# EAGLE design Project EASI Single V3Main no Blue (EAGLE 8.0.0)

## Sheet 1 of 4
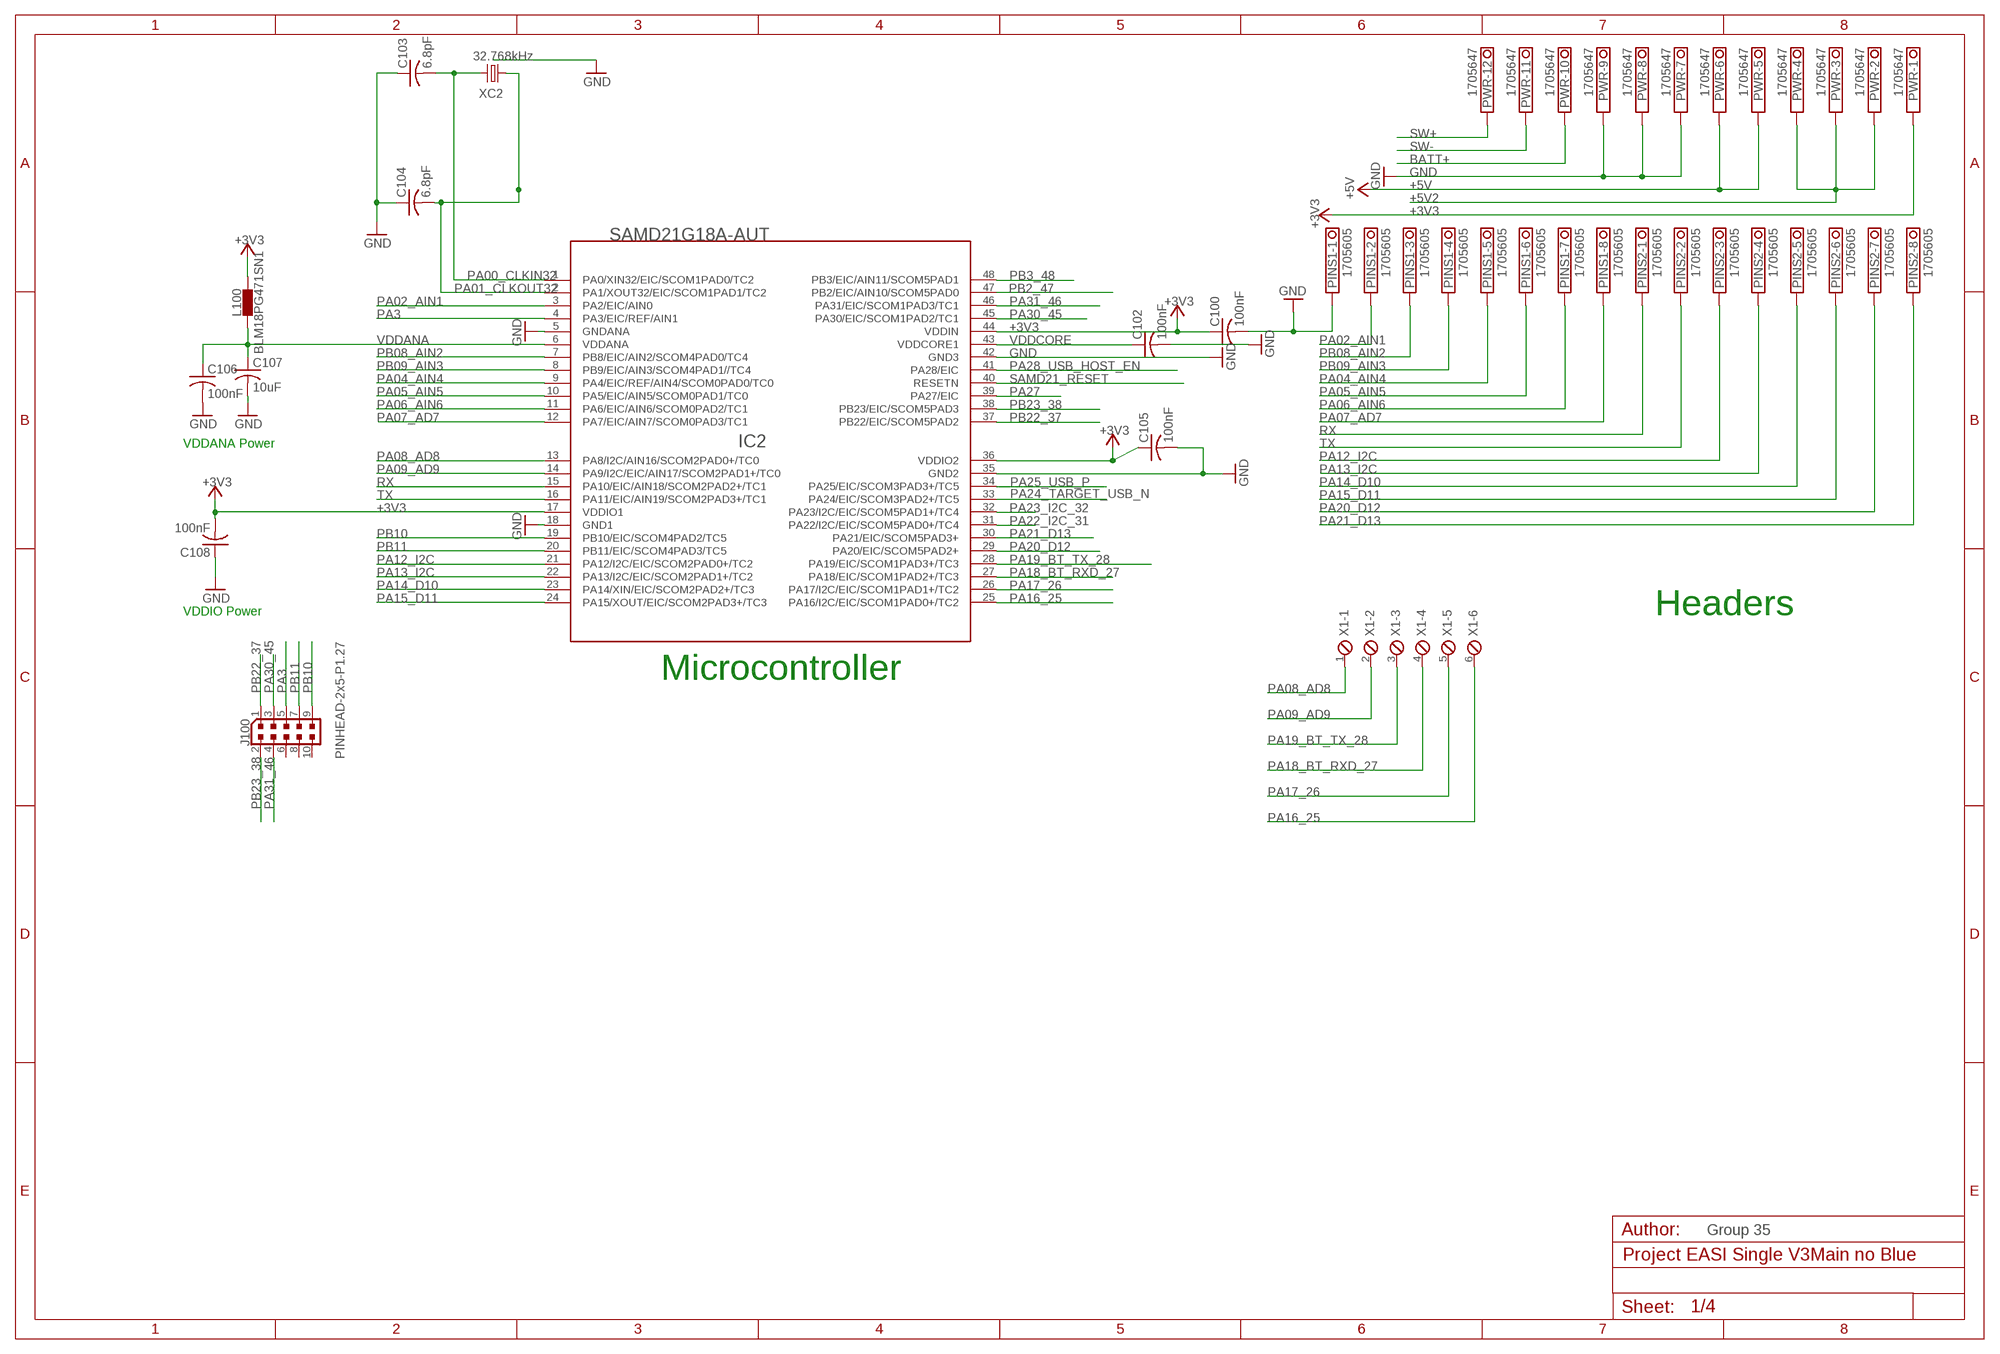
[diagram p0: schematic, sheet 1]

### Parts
C100  100nF  C-USC0805  [C0805]
C102  100nF  C-USC0805  [C0805]
C103  6.8pF  C-USC0805  [C0805]
C104  6.8pF  C-USC0805  [C0805]
C105  100nF  C-USC0805  [C0805]
C106  100nF  C-USC0805  [C0805]
C107  10uF  C-USC0805  [C0805]
C108  100nF  C-USC0805  [C0805]
IC2  SAMD21G18A-AUT  SAMD21G18A  [TQFP48]
J100  PINHEAD-2x5-P1.27  0171_PH127-205DF055G00AROUND-PADS  [PINHEAD_2X05_127]
L100  BLM18PG471SN1  INDUCTOR-0603  [C0603]
PINS1  1705605  [1705605]
PINS2  1705605  [1705605]
PWR  1705647  [1705647]
X1  MPT6  [6POL254]
XC2  32.768kHz  CRYSTALSMD  [CRYSTAL_TC26SMD]

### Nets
+3V3: C100.1 C105.1 C108.2 IC2.17(VDDIO1) IC2.36(VDDIO2) IC2.44(VDDIN) L100.2 PWR.1.1 PWR.1.2 ; also sheet 3
+5V: PWR.5.1 PWR.5.2 PWR.6.1 PWR.6.2 ; also sheet 3
+5V2: PWR.2.1 PWR.2.2 PWR.3.1 PWR.3.2 PWR.4.1 PWR.4.2 ; also sheet 3
BATT+: PWR.10.1 PWR.10.2 ; also sheet 3
GND [gnd]: C100.2 C102.2 C103.1 C104.1 C105.2 C106.2 C107.2 C108.1 IC2.5(GNDANA) IC2.18(GND1) IC2.35(GND2) IC2.42(GND3) PINS1.1.1 PINS1.1.2 PWR.7.1 PWR.7.2 PWR.8.1 PWR.8.2 PWR.9.1 PWR.9.2 XC2.P$1(GND) ; also sheet 3
PA00_CLKIN32: C103.2 IC2.1(PA0/XIN32/EIC/SCOM1PAD0/TC2) XC2.2
PA01_CLKOUT32: C104.2 IC2.2(PA1/XOUT32/EIC/SCOM1PAD1/TC2) XC2.1
PA02_AIN1: IC2.3(PA2/EIC/AIN0) PINS1.2.1 PINS1.2.2
PA3: IC2.4(PA3/EIC/REF/AIN1) J100.5 ; also sheet 2
PA04_AIN4: IC2.9(PA4/EIC/REF/AIN4/SCOM0PAD0/TC0) PINS1.5.1 PINS1.5.2
PA05_AIN5: IC2.10(PA5/EIC/AIN5/SCOM0PAD1/TC0) PINS1.6.1 PINS1.6.2
PA06_AIN6: IC2.11(PA6/EIC/AIN6/SCOM0PAD2/TC1) PINS1.7.1 PINS1.7.2
PA07_AD7: IC2.12(PA7/EIC/AIN7/SCOM0PAD3/TC1) PINS1.8.1 PINS1.8.2
PA08_AD8: IC2.13(PA8/I2C/AIN16/SCOM2PAD0+/TC0) X1.1
PA09_AD9: IC2.14(PA9/I2C/EIC/AIN17/SCOM2PAD1+/TC0) X1.2
PA12_I2C: IC2.21(PA12/I2C/EIC/SCOM2PAD0+/TC2) PINS2.3.1 PINS2.3.2
PA13_I2C: IC2.22(PA13/I2C/EIC/SCOM2PAD1+/TC2) PINS2.4.1 PINS2.4.2
PA14_D10: IC2.23(PA14/XIN/EIC/SCOM2PAD2+/TC3) PINS2.5.1 PINS2.5.2
PA15_D11: IC2.24(PA15/XOUT/EIC/SCOM2PAD3+/TC3) PINS2.6.1 PINS2.6.2
PA16_25: IC2.25(PA16/I2C/EIC/SCOM1PAD0+/TC2) X1.6
PA17_26: IC2.26(PA17/I2C/EIC/SCOM1PAD1+/TC2) X1.5
PA18_BT_RXD_27: IC2.27(PA18/EIC/SCOM1PAD2+/TC3) X1.4
PA19_BT_TX_28: IC2.28(PA19/EIC/SCOM1PAD3+/TC3) X1.3
PA20_D12: IC2.29(PA20/EIC/SCOM5PAD2+) PINS2.7.1 PINS2.7.2
PA21_D13: IC2.30(PA21/EIC/SCOM5PAD3+) PINS2.8.1 PINS2.8.2
PA22_I2C_31: IC2.31(PA22/I2C/EIC/SCOM5PAD0+/TC4) ; also sheet 2
PA23_I2C_32: IC2.32(PA23/I2C/EIC/SCOM5PAD1+/TC4) ; also sheet 2
PA24_TARGET_USB_N [USBpair]: IC2.33(PA24/EIC/SCOM3PAD2+/TC5)
PA25_USB_P [USBpair]: IC2.34(PA25/EIC/SCOM3PAD3+/TC5)
PA27: IC2.39(PA27/EIC)
PA28_USB_HOST_EN: IC2.41(PA28/EIC)
PA30_45: IC2.45(PA30/EIC/SCOM1PAD2/TC1) J100.3 ; also sheet 2
PA31_46: IC2.46(PA31/EIC/SCOM1PAD3/TC1) J100.4 ; also sheet 2
PB2_47: IC2.47(PB2/EIC/AIN10/SCOM5PAD0) ; also sheet 2
PB3_48: IC2.48(PB3/EIC/AIN11/SCOM5PAD1)
PB08_AIN2: IC2.7(PB8/EIC/AIN2/SCOM4PAD0/TC4) PINS1.3.1 PINS1.3.2
PB09_AIN3: IC2.8(PB9/EIC/AIN3/SCOM4PAD1//TC4) PINS1.4.1 PINS1.4.2
PB10: IC2.19(PB10/EIC/SCOM4PAD2/TC5) J100.9
PB11: IC2.20(PB11/EIC/SCOM4PAD3/TC5) J100.7
PB22_37: IC2.37(PB22/EIC/SCOM5PAD2) J100.1
PB23_38: IC2.38(PB23/EIC/SCOM5PAD3) J100.2
RX: IC2.15(PA10/EIC/AIN18/SCOM2PAD2+/TC1) PINS2.1.1 PINS2.1.2
SAMD21_RESET: IC2.40(RESETN) ; also sheet 2
SW+: PWR.12.1 PWR.12.2 ; also sheet 3
SW-: PWR.11.1 PWR.11.2 ; also sheet 3
TX: IC2.16(PA11/EIC/AIN19/SCOM2PAD3+/TC1) PINS2.2.1 PINS2.2.2
VDDANA: C106.1 C107.1 IC2.6(VDDANA) L100.1
VDDCORE: C102.1 IC2.43(VDDCORE1)
Unconnected: J100.6 J100.8 J100.10

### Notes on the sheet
- VDDANA Power
- VDDIO Power | Headers
- Microcontroller
- Group 35

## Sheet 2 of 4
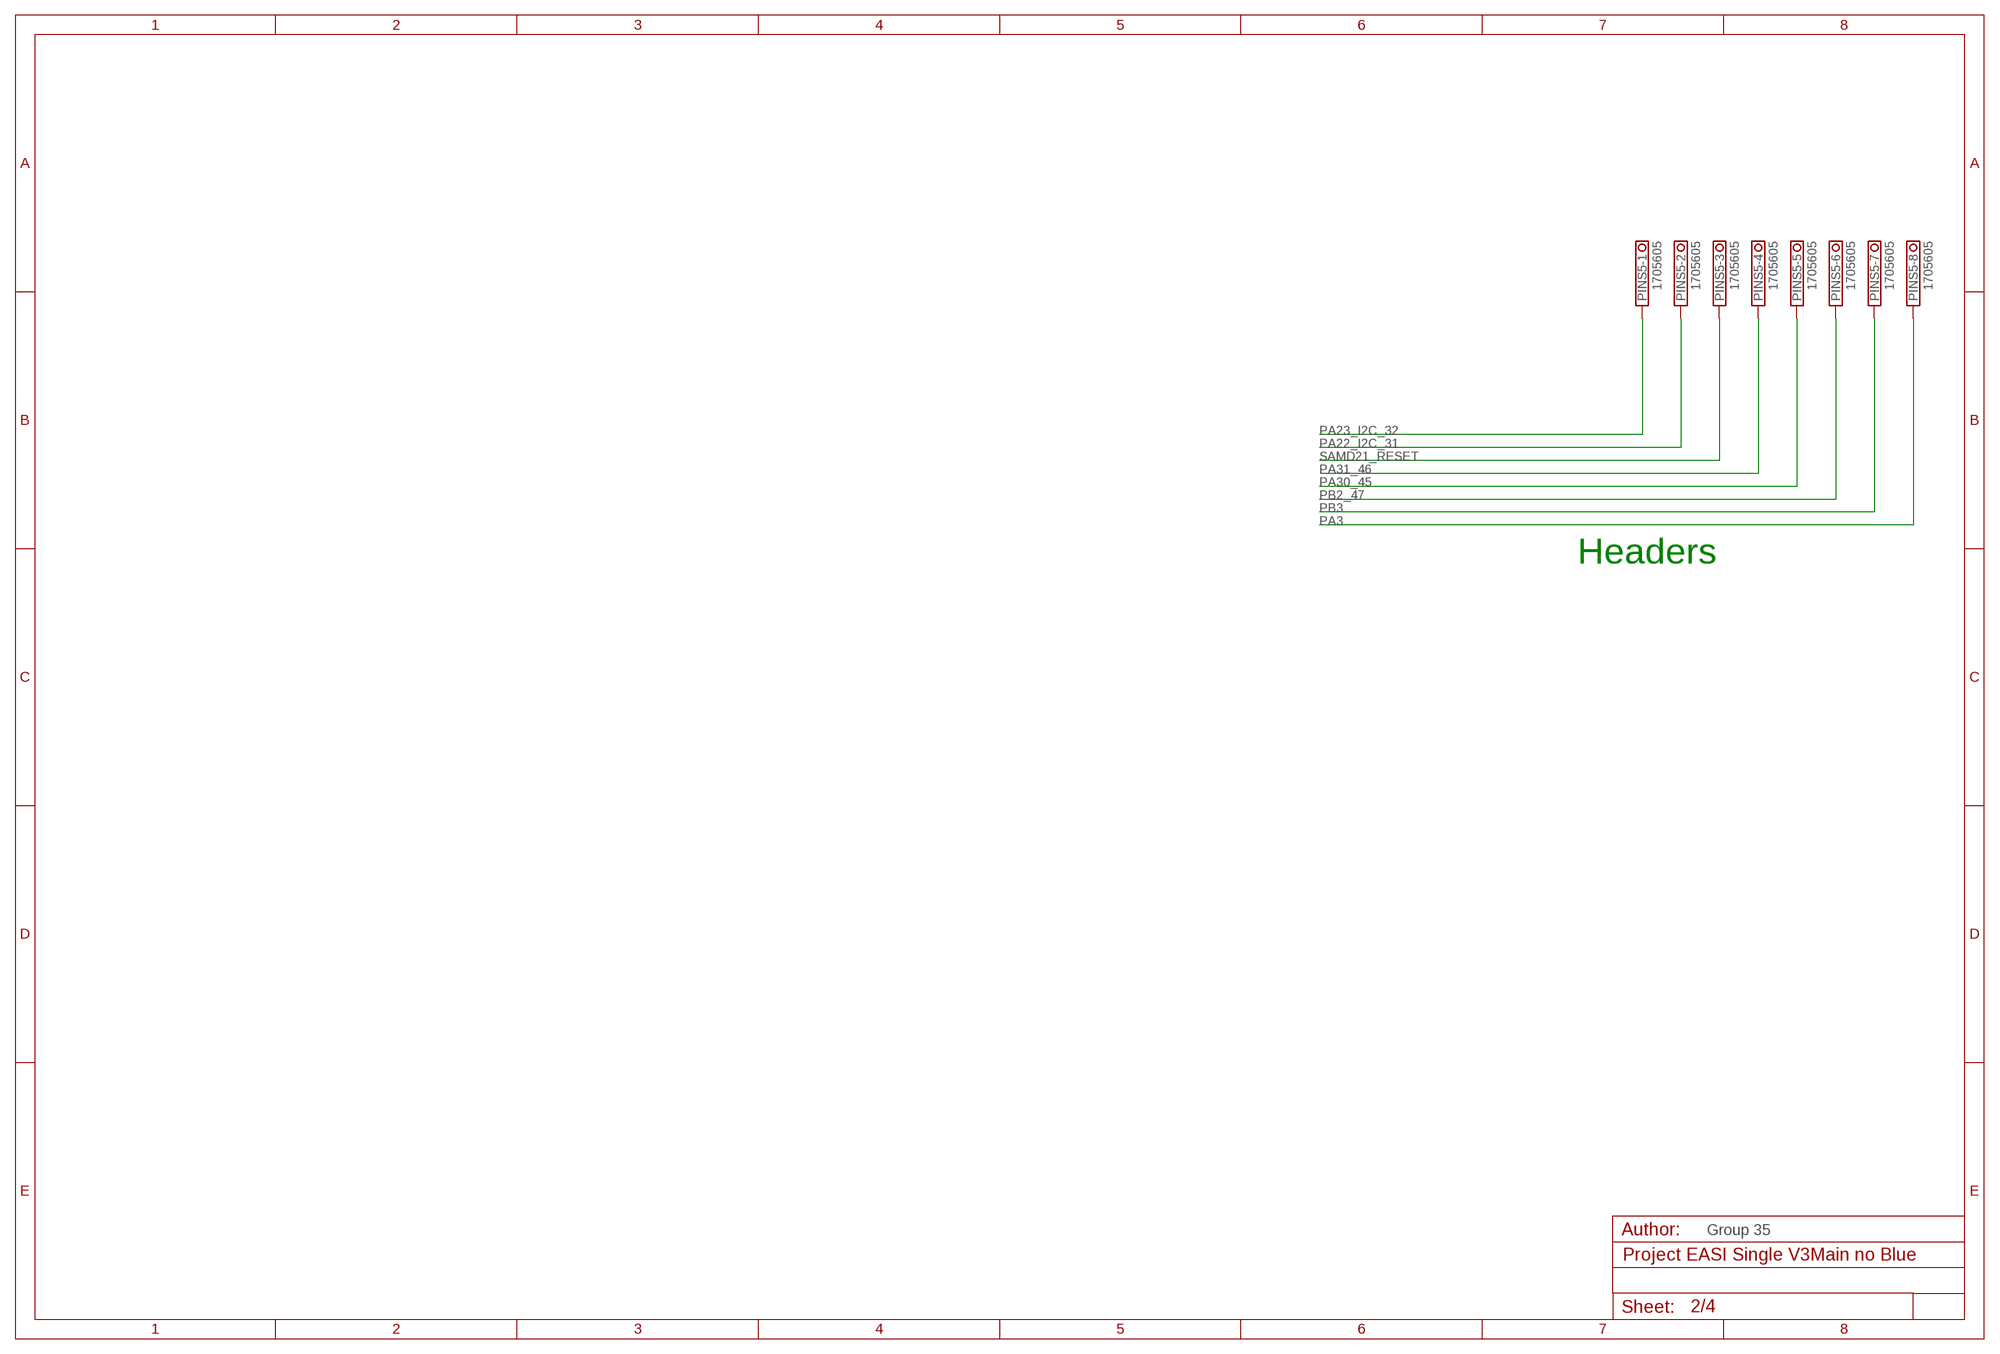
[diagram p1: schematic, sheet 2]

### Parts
PINS5  1705605  [1705605]

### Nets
PA3: PINS5.8.1 PINS5.8.2 ; also sheet 1
PA22_I2C_31: PINS5.2.1 PINS5.2.2 ; also sheet 1
PA23_I2C_32: PINS5.1.1 PINS5.1.2 ; also sheet 1
PA30_45: PINS5.5.1 PINS5.5.2 ; also sheet 1
PA31_46: PINS5.4.1 PINS5.4.2 ; also sheet 1
PB2_47: PINS5.6.1 PINS5.6.2 ; also sheet 1
PB3: PINS5.7.1 PINS5.7.2
SAMD21_RESET: PINS5.3.1 PINS5.3.2 ; also sheet 1

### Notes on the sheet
- Headers
- Group 35

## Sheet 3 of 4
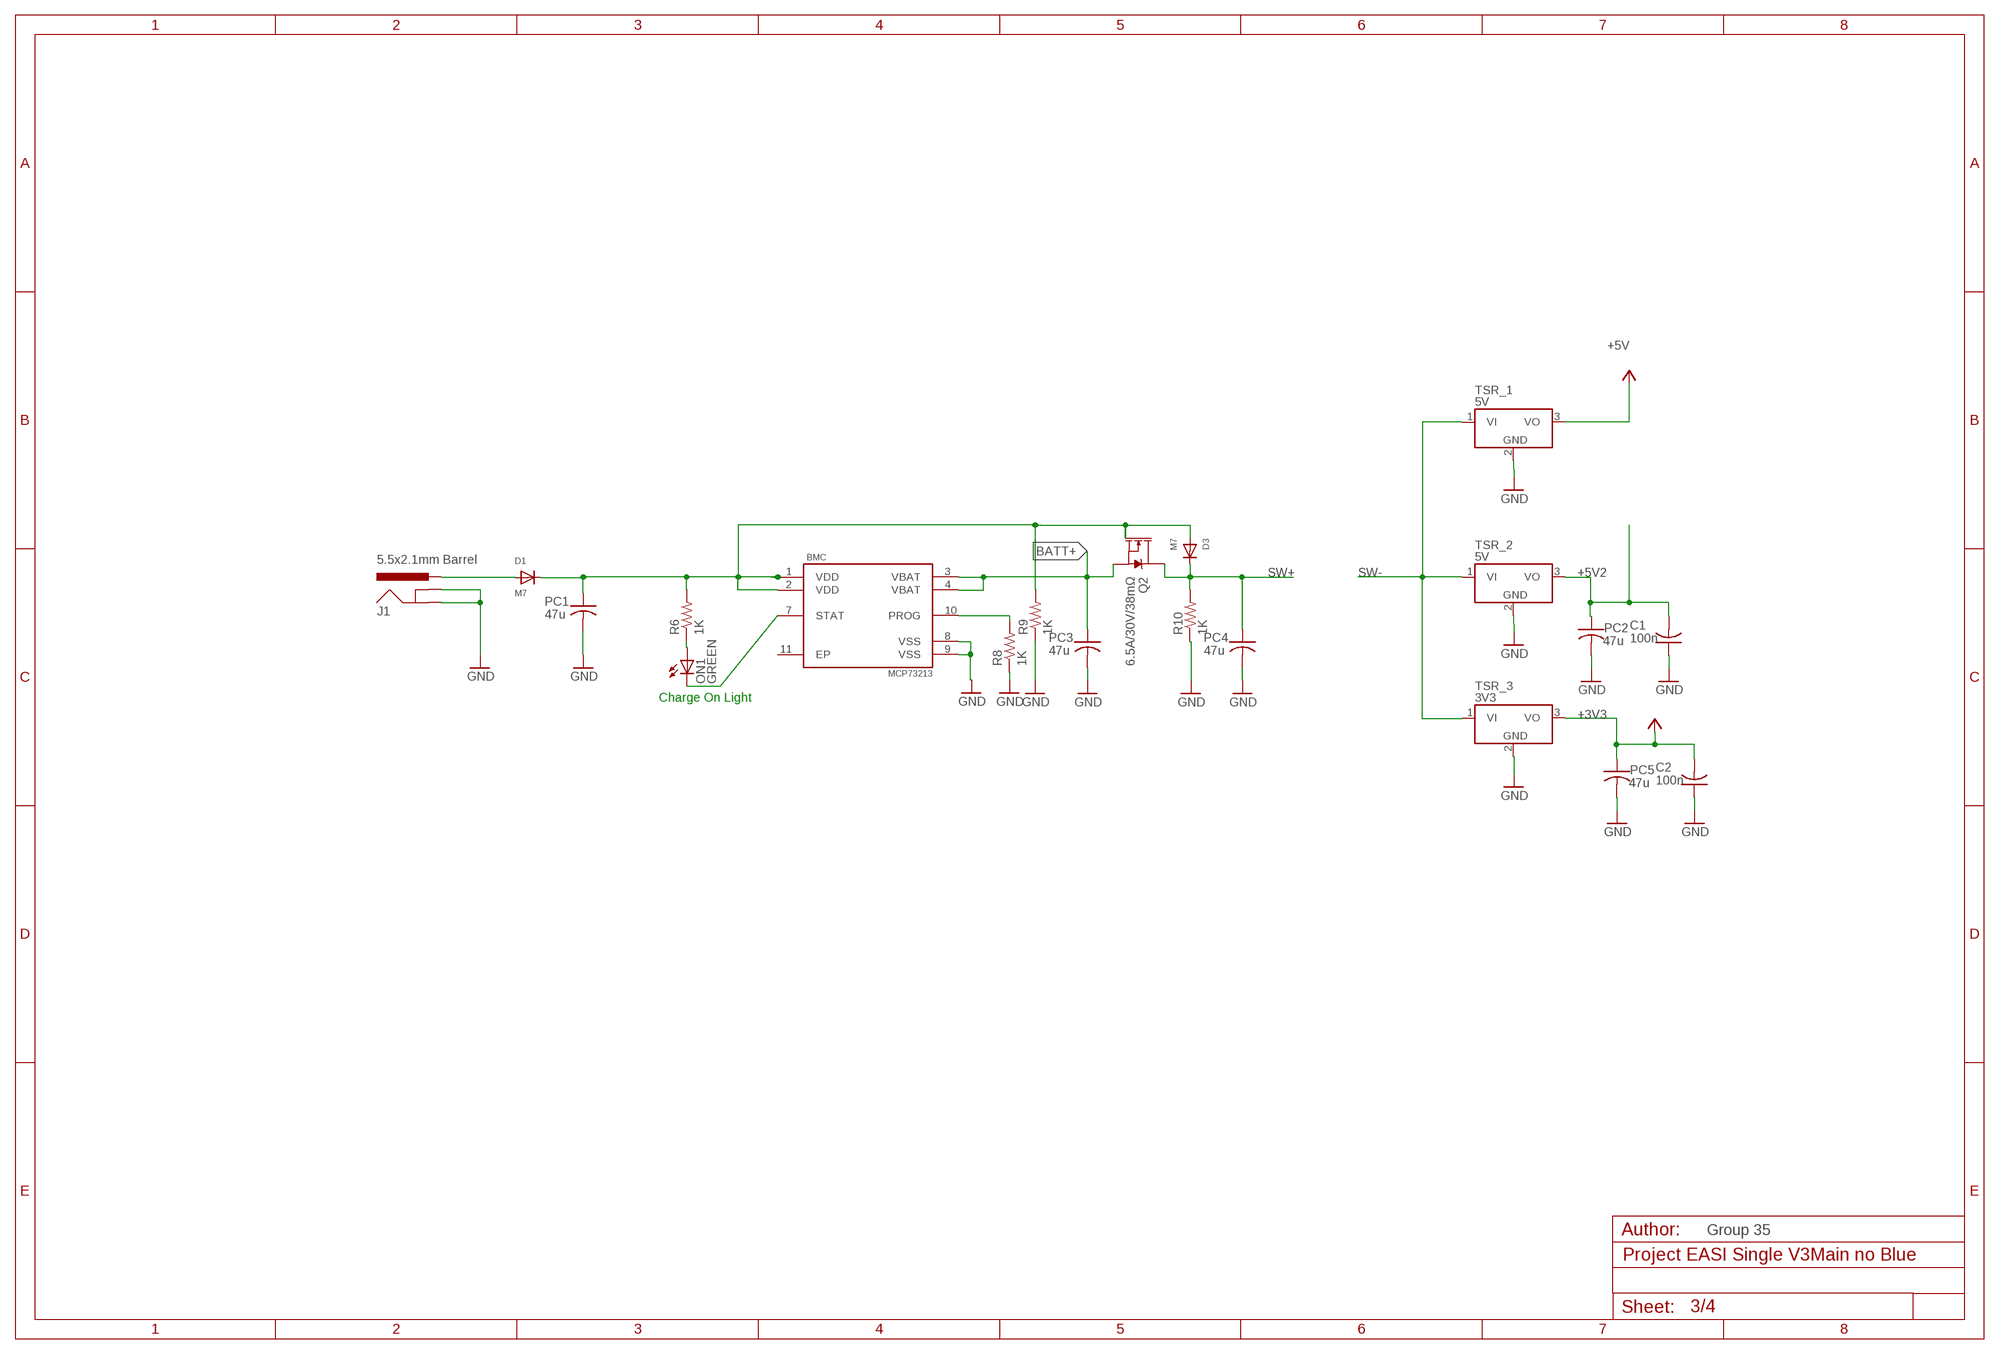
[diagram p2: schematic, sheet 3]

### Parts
BMC  MCP73213  [MCP73213]
C1  100n  C-USC0805  [C0805]
C2  100n  C-USC0805  [C0805]
D1  M7  DIODESMA  [SMADIODE]
D3  M7  DIODESMA  [SMADIODE]
J1  5.5x2.1mm Barrel  POWER_JACKSMD  [POWER_JACK_SMD]
ON1  GREEN  LEDCHIP-LED0805  [CHIP-LED0805]
PC1  47u  C-USC1206  [C1206]
PC2  47u  C-USC1206  [C1206]
PC3  47u  C-USC1206  [C1206]
PC4  47u  C-USC1206  [C1206]
PC5  47u  C-USC1206  [C1206]
Q2  6.5A/30V/38mΩ  MOSFET-NCH-FDS6630A  [SO08]
R6  1K  R-US_R0805  [R0805]
R8  1K  R-US_R0805  [R0805]
R9  1K  R-US_R0805  [R0805]
R10  1K  R-US_R0805  [R0805]
TSR_1  5V  TSR_1-24_  [TSR-1]
TSR_2  5V  TSR_1-24_  [TSR-1]
TSR_3  3V3  TSR_1-24_  [TSR-1]

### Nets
+3V3: C2.2 PC5.1 TSR_3.3(VO) ; also sheet 1
+5V: TSR_1.3(VO) ; also sheet 1
+5V2: C1.2 PC2.1 TSR_2.3(VO) ; also sheet 1
BATT+: BMC.3(VBAT) BMC.4(VBAT) PC3.1 Q2.1(S) Q2.2(S) Q2.3(S) ; also sheet 1
GND [gnd]: BMC.8(VSS) BMC.9(VSS) C1.1 C2.1 J1.GND(GNDBREAK) J1.P$4(GND) PC1.2 PC2.2 PC3.2 PC4.2 PC5.2 R8.1 R9.1 R10.1 TSR_1.2(GND) TSR_2.2(GND) TSR_3.2(GND) ; also sheet 1
N$2: D1.A J1.VIN0(PWR)
N$6: ON1.A R6.1
N$11: BMC.10(PROG) R8.2
N$13: BMC.7(STAT) ON1.C
N$29: BMC.1(VDD) BMC.2(VDD) D1.C D3.A PC1.1 Q2.4(G) R6.2 R9.2
SW+: D3.C PC4.1 Q2.5(D) Q2.6(D) Q2.7(D) Q2.8(D) R10.2 ; also sheet 1
SW-: TSR_1.1(VI) TSR_2.1(VI) TSR_3.1(VI) ; also sheet 1
Unconnected: BMC.11(EP)

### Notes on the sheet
- Charge On Light
- Group 35

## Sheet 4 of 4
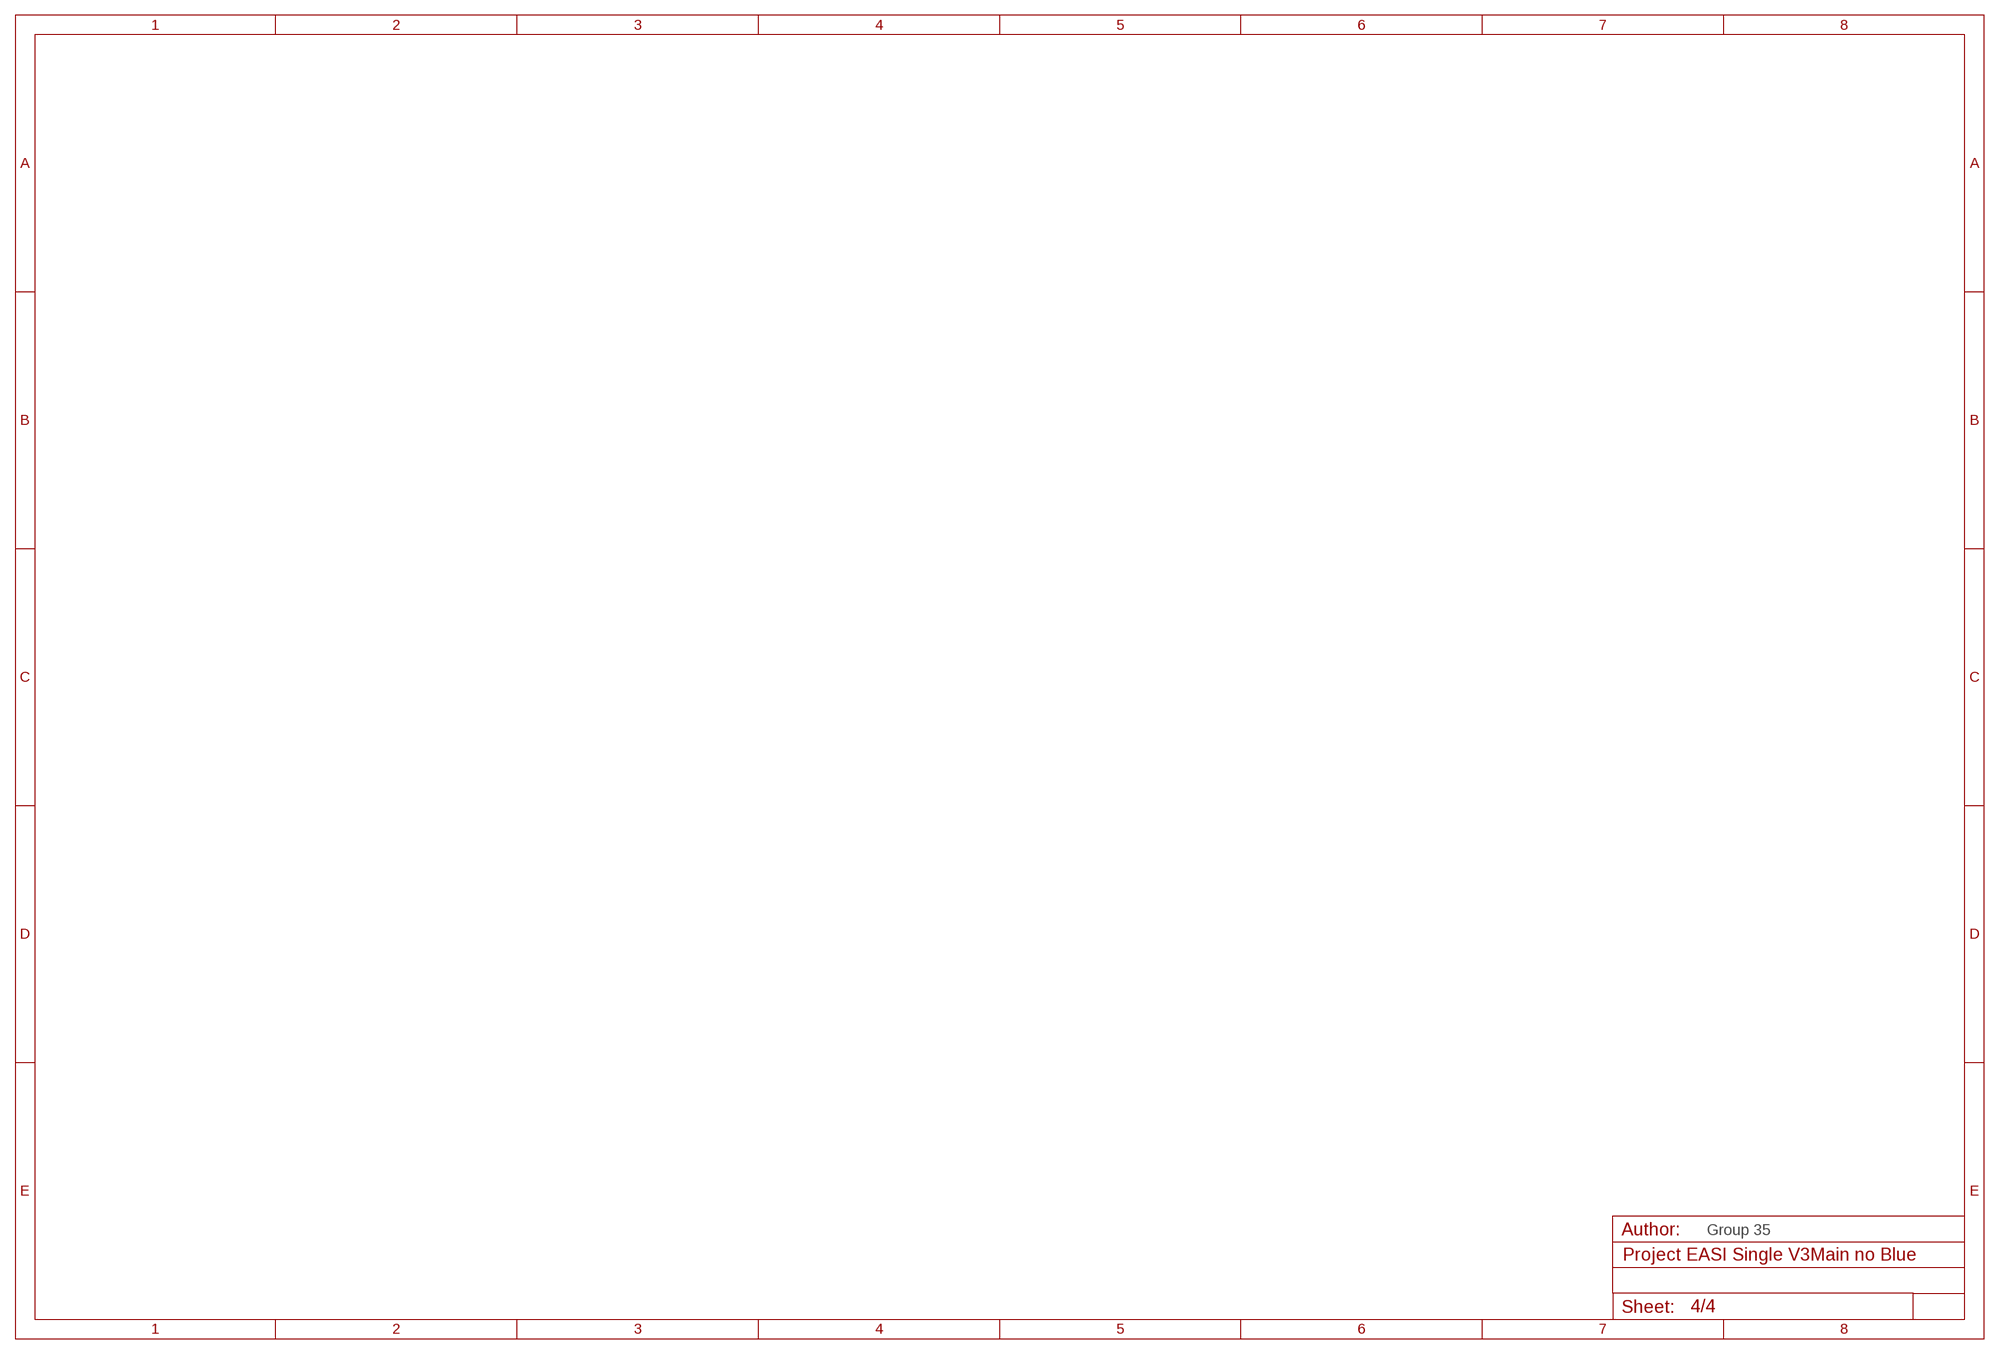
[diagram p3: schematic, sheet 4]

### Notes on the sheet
- Group 35

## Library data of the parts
BMC = Project_EASI_P_DualM_V1:MCP73213; MPN: MCP73213EV-2SOVP; OC_NEWARK: 26R1748
C1 C2 C100 C102-C108 PC1-PC5 = adafruit:C-US: CAPACITOR, American symbol; OC_NEWARK: unknown
D1 D3 = microbuilder:DIODE: Diode; OC_NEWARK: unknown
IC2 = Project_EASI_P_DualM_V1:SAMD21G18A: Atmel D21 32bit ARM Cortex-M0 microcontroller - 48 PIN TQFP 256KB flash memory + 32KB SRAM; OC_NEWARK: unknown
J1 = SparkFun-Connectors:POWER_JACK: Power Jack Connector This is the standard 5.5mm barrel jack for power. The PTH is the most common, proven, reliable, footprint. The Slot footprint only works if the mill layer is transmitted to the PCB fab house so be warned. Here are the connectors we sell at SparkFun: DC Barrel Power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; OC_NEWARK: unknown; PROD_ID: CONN-08106; SF_ID: PRT-12748
J100 = Connettori:0171_PH127-205DF055G00A: 2x5 PASSO 1,27
L100 = Arduino:INDUCTOR: Inductors; OC_NEWARK: unknown
ON1 = led:LED: LED; OC_NEWARK: unknown
PINS1 PINS2 PINS5 = con-phoenix-3.81-bigdrill holes:1705605: MKDSD 1,5/10-3,81 Printklemme Nennstrom: 8 A Bemessungsspannung: 200 V Raster: 3,81 mm Polzahl: 12 Montageart: Löten Anschlussart: Schraubanschluss Anschlussrichtung vom Leiter zur Platine: 0° Source: http://eshop.phoenixcontact.com .. 1705605.pdf; OC_FARNELL: unknown; OC_NEWARK: unknown
PWR = con-phoenix-3.81-bigdrill holes:1705647: MKDSD 1,5/12-3,81 Printklemme Nennstrom: 8 A Bemessungsspannung: 200 V Raster: 3,81 mm Polzahl: 12 Montageart: Löten Anschlussart: Schraubanschluss Anschlussrichtung vom Leiter zur Platine: 0° Source: http://eshop.phoenixcontact.com .. 1705647.pdf; OC_FARNELL: unknown; OC_NEWARK: unknown
Q2 = SparkFun-DiscreteSemi:MOSFET-NCH: N-channel MOSFETs Voltage controlled devices that allow control of high current outputs. SparkFun Products: SparkFun OpenScale SparkFun Digital Sandbox SparkFun Monster Moto Shield SparkFun MOSFET Power Controller; OC_NEWARK: unknown; PROD_ID: TRANS-08089
R6 R8-R10 = adafruit:R-US_: RESISTOR, American symbol; OC_NEWARK: unknown
TSR_1-TSR_3 = _traco_tsr-1:TSR_1-*: TRACO TSR-1 Series Point-of-Load DC/DC-Converters Vi max. 36 V; Vo = (1.2 .. 15)V &plusmn;2%; Io = 0 .. 1 A SIP-Package (drop-in replacement for 78xx linear voltage regulators in TO220-package, vertically assembled) Source: www.tracopower.com Technologies: TSR 1- Vi (V) Vo (V) &plusmn;2% Io = 0 ..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; OC_NEWARK: unknown
X1 = con-phoenix-254:MPT6: PHOENIX CONNECTOR; OC_FARNELL: unknown; OC_NEWARK: unknown
XC2 = Project_EASI_P_DualM_V1:CRYSTAL: Crystals; OC_NEWARK: unknown

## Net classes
0 default: width 0.203 mm, drill 5 mm, clearance 0.203 mm
1 USB: width 0.203 mm, drill 5 mm, clearance 0.203 mm to class 0
2 gnd: width 0.203 mm, drill 5 mm, clearance 0.203 mm to class 0
3 usbvcc: width 0.203 mm, drill 5 mm, clearance 0.203 mm to class 0, clearance 0.15 mm
4 USBpair: width 0.203 mm, drill 5 mm, clearance 0.203 mm to class 0, clearance 0.15 mm to class 3

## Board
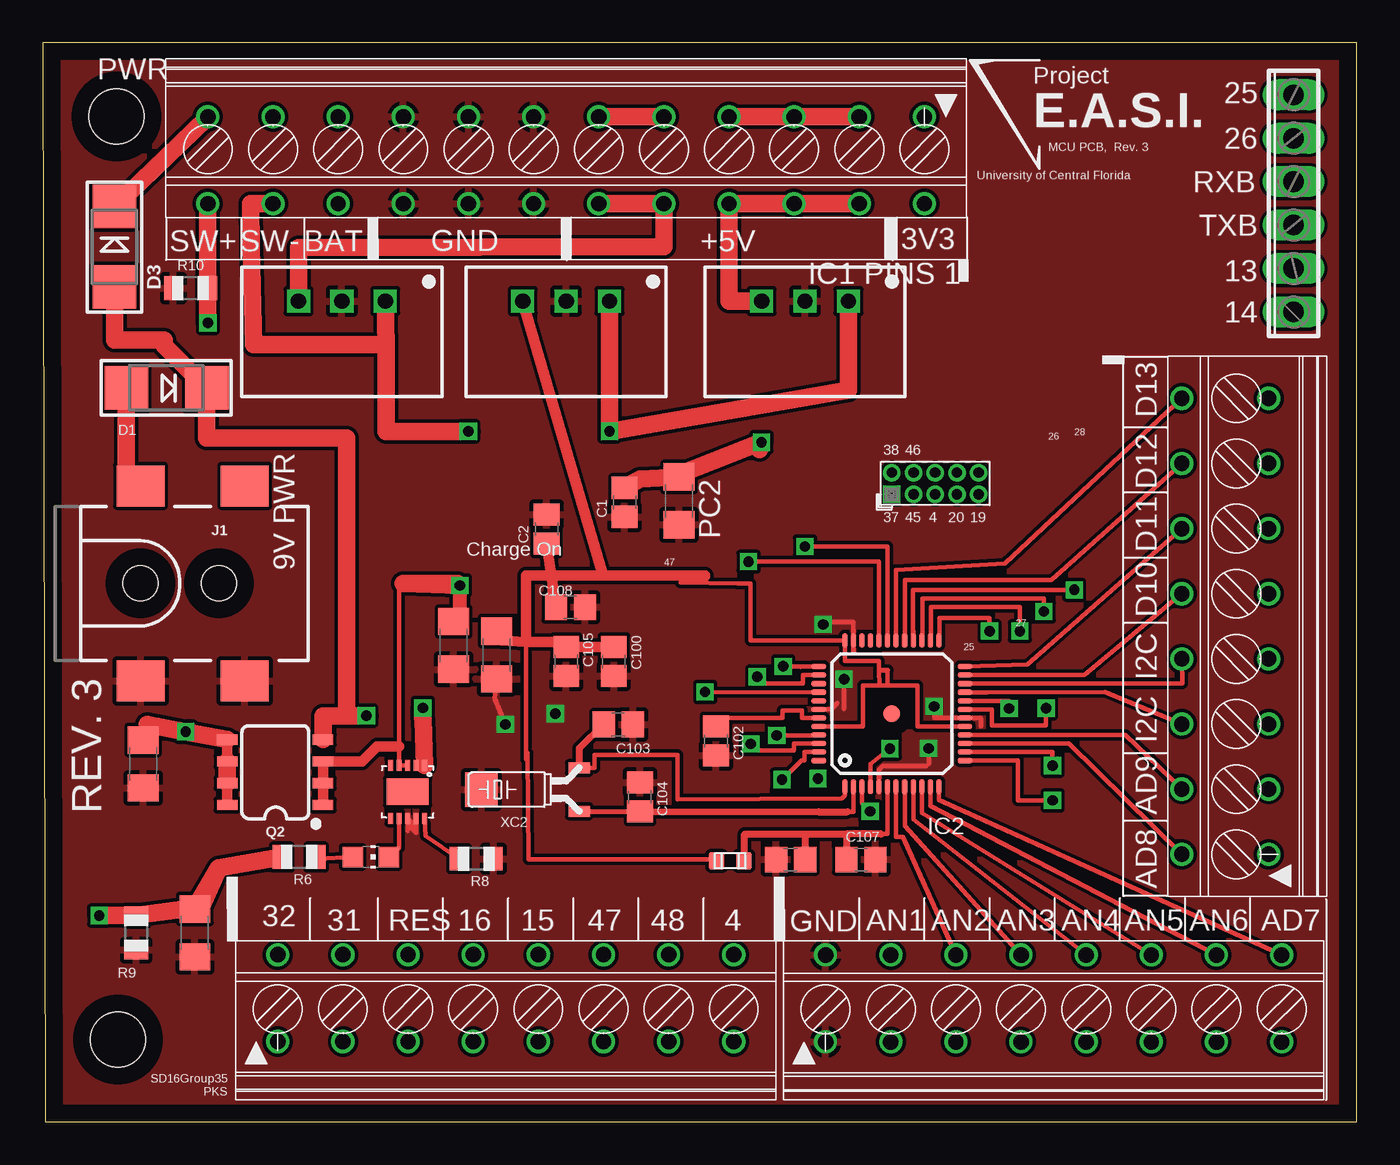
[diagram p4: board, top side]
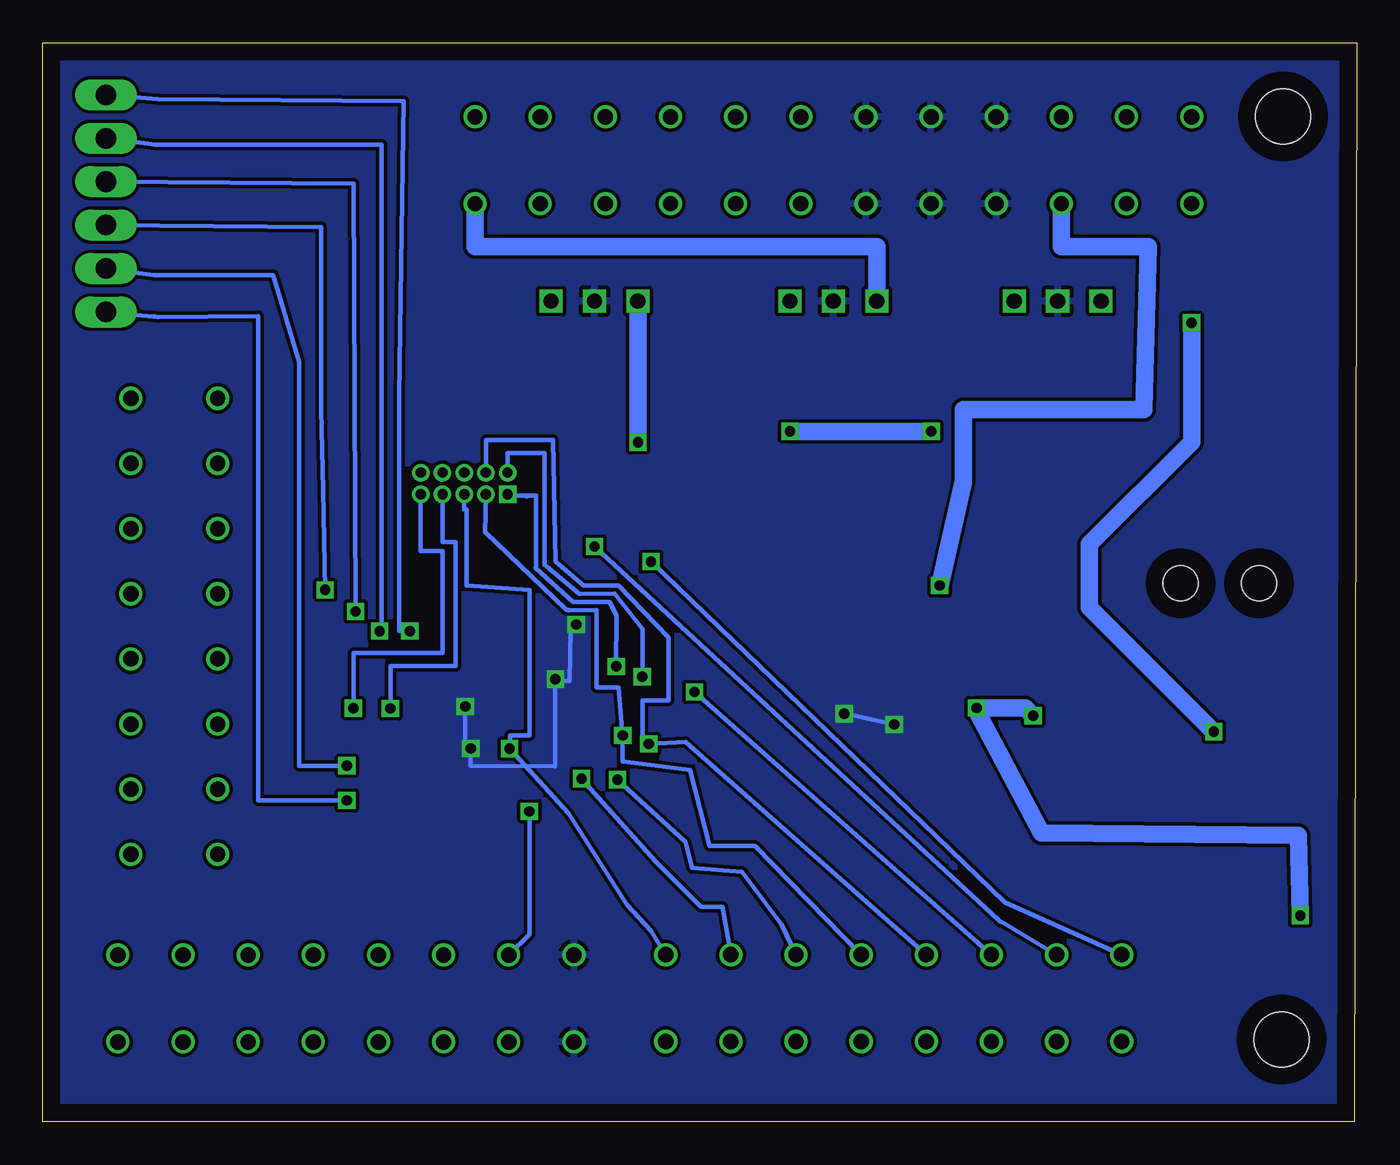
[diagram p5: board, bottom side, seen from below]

Size 76.85 x 63.12 mm. Coordinates in mm from the lower left corner, seen from the top.
Outline: 0.13,0 76.85,0.01 76.85,63.11 0,63.12 0.13,0
Copper layers (1*16): Top 0.035mm / dielectric 1.5mm / Bottom 0.035mm
Design rules "default *": minimum track width 10mil, minimum drill 15mil, track to track 8mil, track to pad 8mil, pad to pad 8mil, via to via 8mil, smd to smd 8mil, copper to edge 40mil, drill to drill 8mil, minimum pad ring 8mil, minimum via ring 8mil, stop-mask expansion 4mil, vias tented up to drill 0mil, thermal gap 10mil
Holes 3.2 mm at 4.39,4.82 4.32,58.8

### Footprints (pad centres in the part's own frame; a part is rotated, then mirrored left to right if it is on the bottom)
MCP73213 = smd 0.65 x 0.3: 1 -1.55,1; 2 -1.55,0.5; 3 -1.55,0; 4 -1.55,-0.5; 5 -1.55,-1; 6 1.55,-1; 7 1.55,-0.5; 8 1.55,0; 9 1.55,0.5; 10 1.55,1 | smd 1.55 x 2.48: 11 0,0
C0805 = smd 1.3 x 1.5: 1 -0.85,0; 2 0.85,0
SMADIODE = smd 2.54 x 2.54: A 2.349,0; C -2.349,0
TQFP48 = smd 0.85 x 0.32: 1 -4.275,2.75; 2 -4.275,2.25; 3 -4.275,1.75; 4 -4.275,1.25; 5 -4.275,0.75; 6 -4.275,0.25; 7 -4.275,-0.25; 8 -4.275,-0.75; 9 -4.275,-1.25; 10 -4.275,-1.75; 11 -4.275,-2.25; 12 -4.275,-2.75; 25 4.275,-2.75; 26 4.275,-2.25; 27 4.275,-1.75; 28 4.275,-1.25; 29 4.275,-0.75; 30 4.275,-0.25; 31 4.275,0.25; 32 4.275,0.75; 33 4.275,1.25; 34 4.275,1.75; 35 4.275,2.25; 36 4.275,2.75 | smd 0.32 x 0.85: 13 -2.75,-4.275; 14 -2.25,-4.275; 15 -1.75,-4.275; 16 -1.25,-4.275; 17 -0.75,-4.275; 18 -0.25,-4.275; 19 0.25,-4.275; 20 0.75,-4.275; 21 1.25,-4.275; 22 1.75,-4.275; 23 2.25,-4.275; 24 2.75,-4.275; 37 2.75,4.275; 38 2.25,4.275; 39 1.75,4.275; 40 1.25,4.275; 41 0.75,4.275; 42 0.25,4.275; 43 -0.25,4.275; 44 -0.75,4.275; 45 -1.25,4.275; 46 -1.75,4.275; 47 -2.25,4.275; 48 -2.75,4.275 | smd 1 x 1: P$1 0,0
POWER_JACK_SMD = smd 2.8 x 2.4: GND 0,-5.7; P$4 6.1,-5.7; VIN0 0,5.7; VIN1 6.1,5.7 | hole 2.032: 0,0; 4.572,0
PINHEAD_2X05_127 = drill 0.6 pad 1.016 square: 1 -0.635,2.54 | drill 0.6 pad 1.016: 2 0.635,2.54; 3 -0.635,1.27; 4 0.635,1.27; 5 -0.635,0; 6 0.635,0; 7 -0.635,-1.27; 8 0.635,-1.27; 9 -0.635,-2.54; 10 0.635,-2.54
C0603 = smd 1 x 0.95: 1 0,0.8; 2 0,-0.8
CHIP-LED0805 = smd 1.2 x 1.2: A 0,-1.05; C 0,1.05
C1206 = smd 1.6 x 1.8: 1 -1.4,0; 2 1.4,0
1705605 = drill 0.9: 1.1 -13.335,-1.25; 1.2 -13.335,3.83; 2.1 -9.525,-1.25; 2.2 -9.525,3.83; 3.1 -5.715,-1.25; 3.2 -5.715,3.83; 4.1 -1.905,-1.25; 4.2 -1.905,3.83; 5.1 1.905,-1.25; 5.2 1.905,3.83; 6.1 5.715,-1.25; 6.2 5.715,3.83; 7.1 9.525,-1.25; 7.2 9.525,3.83; 8.1 13.335,-1.25; 8.2 13.335,3.83
1705647 = drill 0.9: 1.1 -20.955,-1.25; 1.2 -20.955,3.83; 2.1 -17.145,-1.25; 2.2 -17.145,3.83; 3.1 -13.335,-1.25; 3.2 -13.335,3.83; 4.1 -9.525,-1.25; 4.2 -9.525,3.83; 5.1 -5.715,-1.25; 5.2 -5.715,3.83; 6.1 -1.905,-1.25; 6.2 -1.905,3.83; 7.1 1.905,-1.25; 7.2 1.905,3.83; 8.1 5.715,-1.25; 8.2 5.715,3.83; 9.1 9.525,-1.25; 9.2 9.525,3.83; 10.1 13.335,-1.25; 10.2 13.335,3.83; 11.1 17.145,-1.25; 11.2 17.145,3.83; 12.1 20.955,-1.25; 12.2 20.955,3.83
SO08 = smd 0.6 x 1.2: 1 -1.905,-2.8; 2 -0.635,-2.8; 3 0.635,-2.8; 4 1.905,-2.8; 5 1.905,2.8; 6 0.635,2.8; 7 -0.635,2.8; 8 -1.905,2.8
R0805 = smd 1.1 x 1.4: 1 -1,0; 2 1,0
TSR-1 = drill 0.9 square: 1 -2.54,0; 2 0,0; 3 2.54,0
6POL254 = drill 1.2 pad 1.778 long: 1 -6.35,0; 2 -3.81,0; 3 -1.27,0; 4 1.27,0; 5 3.81,0; 6 6.35,0
CRYSTAL_TC26SMD = smd 1.27 x 0.635: 1 0,1.27; 2 0,-1.27 | smd 1.905 x 2.032: P$1 5.715,0

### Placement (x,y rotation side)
BMC  21.34,19.3 270 top
C1  34.03,36.24 90 top
C2  29.47,34.67 270 top
C100  33.41,26.92 270 top
C102  39.38,22.28 270 top
C103  33.66,23.24 180 top
C104  34.93,19 270 top
C105  30.61,26.92 270 top
C106  43.74,15.34 180 top
C107  47.86,15.34 0 top
C108  30.87,30.1 180 top
D1  7.24,42.93 180 top
D3  4.2,51.18 270 top
IC2  49.66,23.88 90 top
J1  5.72,31.5 0 top
J100  52.2,37.34 90 top
L100  40.21,15.27 270 top
ON1  19.18,15.49 270 top
PC1  8.9,11.05 270 top
PC2  37.22,36.32 270 top
PC3  24.03,27.86 270 top
PC4  5.87,20.93 270 top
PC5  26.55,27.3 270 top
PINS1  59.12,5.93 0 top
PINS2  70.45,28.98 90 top
PINS5  27.08,5.94 0 top
PWR  30.61,57.53 180 top
Q2  13.59,20.45 90 top
R6  14.99,15.49 180 top
R8  25.35,15.39 180 top
R9  5.47,11.05 90 top
R10  8.64,48.77 0 top
TSR_1  17.5,48.01 180 top
TSR_2  44.58,48.01 180 top
TSR_3  30.61,48.01 180 top
X1  73.16,53.72 90 top
XC2  31.37,19.43 180 top

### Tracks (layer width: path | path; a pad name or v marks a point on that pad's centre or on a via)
+3V3
  Top 0.254: IC2.44 47.96,23.14 47.96,25.53 48.93,25.53 | 48.93,25.53 51.16,25.53 51.16,23.14 IC2.17 | 48.93,25.53 48.92,26.41 48.92,26.8 48.92,26.95 46.92,26.95 IC2.36 44.91,28.15 42.12,28.15 41.41,28.15 41.41,31.5 40.65,31.5 37.29,31.55 38.74,31.93 | 49.41,26.42 49.41,25.55 48.93,25.53 | 39.32,15.37 39.46,15.37 | 39.46,15.37 39.5,15.34 28.4,15.34 28.35,21.57 28.28,21.18 28.28,28.07 | 39.46,15.37 39.41,15.37 L100.2 | PC5.1 26.55,28.19 26.29,28.19
  Top 0.305: 48.92,26.41 49.41,26.41 49.41,26.42
  Top 0.406: L100.2 arc-90 39.39,15.24
  Top 0.61: TSR_3.3 32.77,31.95 | 30.23,30.19 C108.2 | C108.2 C2.2 | 26.29,28.19 28.28,28.07 | 26.17,28.23 PC5.1 | 28.28,28.07 28.28,31.95 29.81,31.95 | 28.28,28.07 30.61,28.07 C105.1 C100.1 | 32.77,31.95 38.74,31.95 38.74,31.93 | 29.81,31.95 32.77,31.95 | C108.2 29.81,30.1 29.81,31.95
  Bottom 1.016: TSR_3.3 28.07,51.18 51.57,51.18 PWR.1.2
+5V
  Top 1.016: PWR.6.1 PWR.5.1 | TSR_1.3 14.96,51.14 36.33,51.18 PWR.5.2 PWR.6.2
+5V2  (via drill 0.6)
  Top 1.016: 41.92,39.33 v42.04,39.75 37.22,37.85 PC2.1 34.92,37.59 C1.2 | PWR.4.1 PWR.3.1 PWR.2.1 47.76,58.8 | PWR.2.2 PWR.3.2 PWR.4.2 40.14,48.01 TSR_2.3
  Bottom 1.016: TSR_2.3 v42.04,39.75
BATT+  (via drill 0.6)
  Top 0.254: BMC.3 BMC.4 20.84,21.97 20.84,31.47 21.07,31.5
  Top 0.406: v24.39,31.37 24.39,29.62 PC3.1
  Top 0.61: Q2.1 Q2.2 Q2.3 18.67,21.08 19.56,21.97 20.84,21.97
  Top 0.813: 23.68,29.46 24.44,29.36 24.19,28.98 24.39,29.18 v24.39,31.37
  Top 1.016: 24.26,31.5 21.07,31.5 v24.39,31.37 | PC3.1 24.19,29.36 24.44,29.36
  Bottom 1.016: v24.39,31.37 22.99,37.47 22.99,41.66 12.45,41.66 12.2,51.18 17.28,51.18 PWR.10.2
GND  (via drill 0.6)
  Top 0.254: IC2.5 48.91,20.59 49.14,20.81 51.69,20.81 51.82,20.94 v51.82,21.84 | IC2.42 46.1,24.13 46.49,24.51 | 47.41,27.52 IC2.35 47.43,28.15 47.43,29.23 46.03,29.23 v45.65,29.08 | v46.87,25.88 46.87,24.16 | IC2.18 | PC5.2 26.42,24.76 v27.06,23.24 | 53.35,23.63 IC2.18 | 53.35,23.63 52.21,23.63 52.2,23.62 52.2,24.23 v52.14,24.29 52.14,23.63 53.35,23.63 | IC2.18 53.35,23.63 | 21.84,16.9 BMC.9 | 21.84,16.9 21.85,16.89 21.85,17.25 BMC.8 21.34,17.02 | 21.34,17.4 21.84,16.9 | 53.35,23.63 53.35,23.62 54.23,23.62 | 54.23,23.62 54.87,23.62 54.87,23.11 | IC2.18 54.23,23.62 | IC2.18 53.35,23.63
  Bottom 0.254: 46.89,25.86 46.89,20.78 51.82,20.82 v51.82,21.84 52.14,22.16 v52.14,24.29 | v45.65,29.08 45.65,29.03 45.98,28.7 46.04,25.78 46.87,25.78 | v27.06,23.24 v29.98,23.88
  pour Bottom: -4.95,83.82 148.72,83.82 148.72,-3.81 -4.95,-3.81
  pour Top: -8.76,86.36 169.04,86.36 169.04,-8.89 -8.76,-8.89
N$2
  Top 1.016: D1.A 4.9,38.02 J1.VIN0
N$6
  Top 0.254: ON1.A 16.12,15.37 R6.1
N$11
  Top 0.254: BMC.10 22.39,16.74 R8.2
N$13
  Top 0.254: BMC.7 20.84,16.03 ON1.C
N$29  (via drill 0.6)
  Top 0.254: BMC.2 BMC.1
  Top 1.016: v22.23,24.21 22.23,23.62 22.26,23.52 BMC.1 | v3.31,12.06 5.47,12.06 | 5.47,12.06 R9.2 | 5.47,12.06 9.28,12.57 | 9.28,12.57 10.29,14.86 | 10.29,14.86 PC1.1 | 9.28,12.57 9.02,12.45 10.29,14.86 | 10.29,14.86 R6.2 | 17.79,23.75 v18.93,23.75 | 17.79,23.75 16.39,23.75 Q2.4 | D3.A 4.2,45.72 7.12,45.72 7.12,45.4 D1.C 9.59,40.01 17.79,40.01 17.79,23.75
  Bottom 1.016: v3.31,12.06 3.43,16.76 18.45,16.89 22.23,24 v22.23,24.21 19.39,24.21 v18.93,23.75
PA00_CLKIN32
  Top 0.254: XC2.2 32.26,20.7 32.26,21.46 37.14,21.46 37.14,18.87 46.74,18.92 46.91,19.09 IC2.1
  Top 0.406: C103.2 31.37,21.84 XC2.2
PA01_CLKOUT32
  Top 0.254: 47.07,18.14 47.41,18.14 IC2.2
  Top 0.305: XC2.1 35.18,18.16
  Top 0.406: 35.18,18.16 C104.2 45.37,18.14 47.07,18.14
PA02_AIN1  (via drill 0.6)
  Top 0.254: IC2.3 47.91,18.64 v48.39,18.16
  Bottom 0.254: v48.39,18.16 48.39,10.96 PINS1.2.2
PA3  (via drill 0.6)
  Top 0.254: IC2.4 48.42,20.37 48.41,20.37 48.41,20.72 48.42,20.95 v49.56,21.83
  Bottom 0.254: J100.5 52.2,35.81 52.08,35.81 52.08,31.37 48.39,31.11 48.39,22.61 49.54,22.61 49.54,21.45 v49.56,21.83 46.11,18.03 42.68,12.7 41.28,11.18 PINS5.8.2
PA04_AIN4
  Top 0.254: IC2.9 50.91,17.68 PINS1.5.2
PA05_AIN5
  Top 0.254: IC2.10 51.42,18.06 PINS1.6.2
PA06_AIN6
  Top 0.254: IC2.11 | IC2.11 51.91,18.49 PINS1.7.2
PA07_AD7
  Top 0.254: IC2.12 52.42,18.82 PINS1.8.2
PA08_AD8  (via drill 0.6)
  Top 0.254: IC2.13 57.03,21.13 57.03,18.8 v59.06,18.8
  Bottom 0.254: v59.06,18.8 64.27,18.8 64.27,47.12 70.11,47.08 | 70.11,47.08 70.36,47.12 | 70.11,47.08 X1.1
PA09_AD9  (via drill 0.6)
  Top 0.254: 54.18,21.61 IC2.14 59.06,21.63 v59.06,20.83
  Bottom 0.254: v59.06,20.83 61.85,20.83 61.85,44.45 63.38,49.53 70.36,49.53 X1.2
PA12_I2C
  Top 0.254: IC2.21 55.25,25.13 62.11,25.15 PINS2.3.2
PA13_I2C
  Top 0.254: IC2.22 66.66,25.63 PINS2.4.2
PA14_D10
  Top 0.254: IC2.23 60.91,26.13 PINS2.5.2
PA15_D11
  Top 0.254: IC2.24 57.6,26.75 PINS2.6.2
PA16_25  (via drill 0.6)
  Top 0.254: IC2.25 52.46,28.15 52.46,29.46 55.38,29.46 v55.38,28.7
  Bottom 0.254: v55.38,28.7 56.01,28.7 56.01,42.42 55.76,59.69 70.11,59.82 X1.6
PA17_26  (via drill 0.6)
  Top 0.254: IC2.26 51.95,28.15 51.95,30.1 57.16,30.1 v57.16,28.7
  Bottom 0.254: v57.16,28.7 57.03,28.7 57.03,40.26 | 57.03,40.26 57.03,40.77 | 57.03,40.64 57.03,41.15 | 57.03,41.15 57.03,57.15 70.24,57.15 X1.5 | 57.03,41.15 57.03,40.26
PA18_BT_RXD_27  (via drill 0.6)
  Top 0.254: IC2.27 51.44,28.15 51.44,30.61 58.55,30.61 v58.55,29.84
  Bottom 0.254: X1.4 58.68,54.86 v58.55,29.84
PA19_BT_TX_28  (via drill 0.6)
  Top 0.254: IC2.28 50.91,28.7 | 50.91,28.7 50.91,31.11 v60.33,31.11 | 50.91,28.7 IC2.28
  Bottom 0.254: v60.33,31.11 60.46,36.96 60.58,41.66 60.58,52.32 X1.3
PA20_D12
  Top 0.254: IC2.29 50.42,28.15 50.42,31.7 58.99,31.7 PINS2.7.2
PA21_D13
  Top 0.254: IC2.30 49.91,32.28 56.27,32.66 PINS2.8.2
PA22_I2C_31  (via drill 0.6)
  Top 0.254: IC2.31 49.41,33.66 v44.58,33.66
  Bottom 0.254: v44.58,33.66 20.97,11.8 | 20.97,11.8 20.83,11.68 | 20.97,11.8 PINS5.2.2
PA23_I2C_32  (via drill 0.6)
  Top 0.254: IC2.32 48.91,32.77 v41.28,32.77
  Bottom 0.254: v41.28,32.77 20.58,12.83 PINS5.1.2
PA25_USB_P
  Top 0.254: IC2.34
PA30_45  (via drill 0.6)
  Top 0.254: IC2.45 45.39,22.61 v42.93,22.61
  Bottom 0.254: J100.3 50.99,34.51 46.23,29.97 46.22,29.96 46.23,29.95 46.06,29.93 46.06,29.92 44.45,29.94 44.46,25.4 43.19,25.4 v42.93,22.61 42.93,21.08 38.99,20.57 37.85,16.13 35.18,16.13 PINS5.5.2
PA31_46  (via drill 0.6)
  Top 0.254: IC2.46 43.95,22.13 43.95,21.72 41.66,21.72 v41.41,22.1
  Bottom 0.254: J100.4 50.93,39.88 47,39.88 46.87,32.77 45.22,31.37 43.19,31.37 40.26,28.32 40.26,24.64 41.79,24.64 41.79,22.1 v41.41,22.1 39.25,22.23 PINS5.4.2
PB2_47  (via drill 0.6)
  Top 0.254: IC2.47 44.56,21.63 44.56,21.14 44.37,21.14 v43.24,20.01
  Bottom 0.254: v43.24,20.01 39.25,16.38 38.87,14.86 35.95,14.61 33.66,11.56 PINS5.6.2
PB3  (via drill 0.6)
  Bottom 0.254: v45.34,20.07 41.03,15.24 38.36,12.57 37.09,12.57 PINS5.7.2
PB08_AIN2
  Top 0.254: IC2.7 49.91,16.66 50.3,16.66 PINS1.3.2
PB09_AIN3
  Top 0.254: IC2.8 50.42,17.3 PINS1.4.2
PB10  (via drill 0.6)
  Top 0.254: IC2.19 55.5,24.13 55.5,23.18 58.68,23.18 v58.68,24.19
  Bottom 0.254: v58.68,24.19 58.68,27.43 53.47,27.43 53.47,33.4 54.74,33.4 J100.9
PB11  (via drill 0.6)
  Top 0.254: IC2.20 56.52,24.63 v56.52,24.18
  Bottom 0.254: v56.52,24.18 56.52,26.67 52.71,26.67 52.71,33.91 53.47,33.91 J100.7
PB22_37  (via drill 0.6)
  Top 0.254: IC2.37 44.46,26.63 | 44.46,26.63 44.31,26.62 | 44.46,26.63 43.94,26.63 v43.31,26.64
  Bottom 0.254: v43.31,26.64 43.31,29.63 43.71,30.41 45.83,30.41 48.03,32.4 48,32.47 48,36.62 48.55,36.62 | 48.55,36.62 48.55,36.59 | 48.55,36.62 49.66,36.62 J100.1
PB23_38  (via drill 0.6)
  Top 0.254: IC2.38 44.46,26.13 44.46,25.65 41.92,25.65 v41.79,26.04
  Bottom 0.254: v41.79,26.04 41.79,28.83 43.42,30.89 45.46,30.87 47.23,32.38 47.25,32.38 | 47.49,32.58 47.25,32.38 | 47.25,32.38 47.49,32.58 | 47.49,32.58 47.5,39.12 49.66,39.12 J100.2
RX
  Top 0.254: IC2.15 60.02,22.13 PINS2.1.2
SAMD21_RESET  (via drill 0.6)
  Top 0.254: 45.39,25.15 IC2.40 v38.74,25.15
  Bottom 0.254: v38.74,25.15 PINS5.3.2
SW+  (via drill 0.6)
  Top 0.61: Q2.8 Q2.6 Q2.5
  Top 1.016: PWR.12.2 9.64,53.7 R10.2 | R10.2 9.64,47.37 | Q2.7 Q2.6 | Q2.5 v8.35,22.81 6.1,23.24 6.1,22.33 PC4.1 | PWR.12.1 arc-90 9.55,58.67 D3.C | R10.2 9.64,46.75 v9.66,46.74
  Bottom 1.016: v9.66,46.74 9.66,39.75 15.63,33.78 15.63,30.09 v8.35,22.81
SW-  (via drill 0.6)
  Top 1.016: TSR_1.1 20.07,45.47 | 20.07,45.47 12.32,45.47 12.2,51.18 12.17,53.7 PWR.11.2 | 20.07,45.47 20.07,40.39 v24.9,40.39 | TSR_3.1 v33.15,40.39 47.12,42.8 TSR_2.1
  Bottom 1.016: v24.9,40.39 v33.15,40.39
TX
  Top 0.254: 53.94,22.64 IC2.16 63.33,22.63 PINS2.2.2
VDDANA
  Top 0.254: IC2.6 49.41,16.84 49.05,16.84
  Top 0.406: L100.1 41.05,15.27 41.05,16.84 44.59,16.84 | 44.59,16.84 C106.1 | 44.59,16.84 47.01,16.84 | 47.01,16.84 C107.1 | 49.05,16.84 47.01,16.84
VDDCORE
  Top 0.254: IC2.43 44.4,23.62 44.4,24.05 43.26,24.05 43.26,23.62 40.01,23.62 40.01,23.37 39.38,23.37 C102.1

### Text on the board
tPlace: Project | 25 | E.A.S.I. | 26 | MCU PCB, Rev. 3 | RXB | University of Central Florida | TXB | SW+ | SW- | BAT | GND | +5V | 3V3 | 13 | IC1 PINS 1 | 14 | D13 | 26 | 28 | 38 | 46 | D12 | 37 | 45 | 4 | 20 | 19 | 47 | D11 | 9V PWR | D10 | 27 | 25 | I2C | I2C | REV. 3 | AD9 | AD8 | 32 | 31 | RES | 16 | 15 | 47 | 48 | 4 | GND | AN1 | AN2 | AN3 | AN4 | AN5 | AN6 | AD7 | SD16Group35 / PKS
tSilk: Charge On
